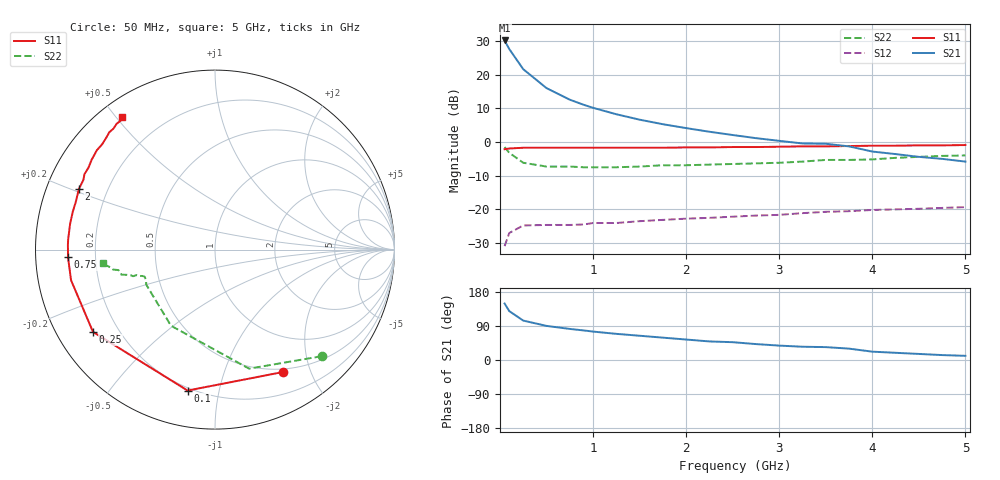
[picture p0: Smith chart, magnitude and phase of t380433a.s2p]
!AT-38043
!S-PARAMETERS at Vce=3.0V Ic=50mA. LAST UPDATED 01-06-98
# ghz s ma r 50
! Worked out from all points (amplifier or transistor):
!   23 points, 50 MHz to 5 GHz, reference 50 ohm
!   highest |S21| = 30.3 dB at 50 MHz (marker M1)
!   |S21| within 3 dB of that: start of sweep to 111.1 MHz
!   unconditionally stable (mu >= 1): 1.537 GHz to end of sweep
!   at 500 MHz: K = 0.40, MSG = 20.4 dB, |S12| = -24.7 dB
!   at 2.25 GHz: K = 1.25, MAG = 9.8 dB, |S12| = -22.6 dB
!   at 5 GHz: K = 1.22, MAG = 3.9 dB, |S12| = -19.4 dB
!   S11 on the Smith chart (normalised r, x): 50 MHz: 0.46, -1.60; 100 MHz: 0.19, -0.81; 250 MHz: 0.11, -0.30; 750 MHz: 0.10, -0.03; 2 GHz: 0.10, +0.21; 5 GHz: 0.07, +0.52
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0.05  0.78 -61.0  32.58 149.0  0.028 55.0  0.84 -45.0
0.1  0.8 -101.0  24.27 129.0  0.044 42.0  0.69 -74.0
0.25  0.82 -146.0  12.16 104.0  0.057 25.0  0.49 -120.0
0.5  0.82 -168.0  6.35 90.0  0.058 22.0  0.43 -145.0
0.75  0.82 -177.0  4.27 82.0  0.058 21.0  0.43 -153.0
0.9  0.82 178.0  3.58 78.0  0.059 21.0  0.42 -156.0
1  0.82 176.0  3.23 75.0  0.062 23.0  0.42 -157.0
1.25  0.82 170.0  2.59 69.0  0.062 26.0  0.42 -159.0
1.5  0.82 165.0  2.15 64.0  0.066 27.0  0.43 -160.0
1.75  0.82 161.0  1.84 59.0  0.069 29.0  0.45 -161.0
2  0.83 156.0  1.61 54.0  0.072 34.0  0.45 -161.0
2.25  0.83 152.0  1.42 49.0  0.074 36.0  0.46 -162.0
2.5  0.84 150.0  1.27 47.0  0.077 29.0  0.47 -162.0
2.75  0.84 147.0  1.14 42.0  0.08 40.0  0.48 -162.0
3  0.85 144.0  1.04 38.0  0.082 42.0  0.49 -163.0
3.25  0.86 140.0  0.95 35.0  0.087 43.0  0.51 -164.0
3.5  0.86 137.0  0.94 34.0  0.091 44.0  0.54 -165.0
3.75  0.87 134.0  0.86 30.0  0.093 45.0  0.54 -166.0
4  0.88 132.0  0.72 22.0  0.097 45.0  0.55 -168.0
4.25  0.88 130.0  0.66 19.0  0.099 45.0  0.58 -169.0
4.75  0.89 126.0  0.56 13.0  0.104 45.0  0.62 -172.0
5  0.9 125.0  0.51 11.0  0.107 46.0  0.63 -173.0
